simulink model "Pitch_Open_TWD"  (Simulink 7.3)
settings: Solver=ode45  StartTime=0.0  StopTime=20  RelTol=1e-3
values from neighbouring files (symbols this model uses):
  Aac = [    [actuator_srb.m]    (also in actuator_ssme.m; actuators_5s.m; actuators_5z.m)
  Bac = [    [actuator_srb.m]    (also in actuator_ssme.m; actuators_5s.m; actuators_5z.m)
  Cac = [    [actuator_srb.m]    (also in actuator_ssme.m; actuators_5s.m; actuators_5z.m)
  Dac = [    [actuator_srb.m]    (also in actuator_ssme.m; actuators_5s.m; actuators_5z.m)
undefined symbols (not defined in the file or in its folder): Afs, Asb, Atw, Bfs, Bsb, Btw, Cfs, Csb, Ctw, Dfs, Dsb, Dtw

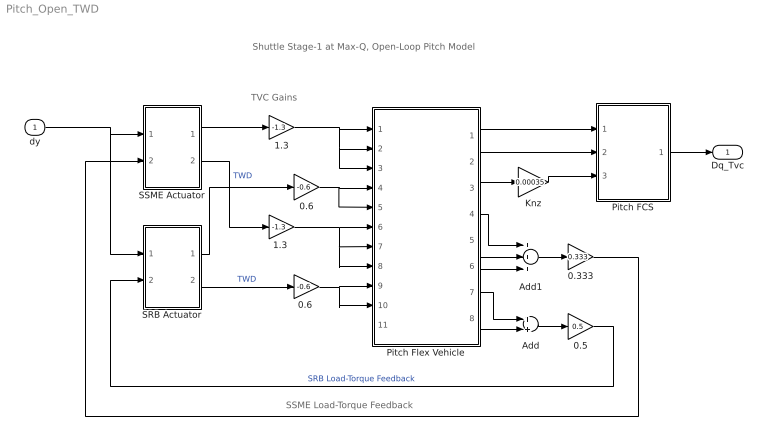
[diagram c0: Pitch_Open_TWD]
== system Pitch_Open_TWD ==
  note: SSME Load-Torque Feedback
  note: TVC Gains
  note: Shuttle Stage-1 at Max-Q, Open-Loop Pitch Model
  dy : Inport  OutDataType=sfix(16)  OutScaling=2^0
  0.333 : Gain  Gain=0.333  ParameterDataType=sfix(16)  ParameterScaling=2^0  OutDataType=sfix(16)  OutScaling=2^0
  0.5 : Gain  Gain=0.5  ParameterDataType=sfix(16)  ParameterScaling=2^0  OutDataType=sfix(16)  OutScaling=2^0
  0.6 : Gain  Gain=-0.6  ParameterDataType=sfix(16)  ParameterScaling=2^0  OutDataType=sfix(16)  OutScaling=2^0
  "0.6 " : Gain  Gain=-0.6  ParameterDataType=sfix(16)  ParameterScaling=2^0  OutDataType=sfix(16)  OutScaling=2^0
  1.3 : Gain  Gain=-1.3  ParameterDataType=sfix(16)  ParameterScaling=2^0  OutDataType=sfix(16)  OutScaling=2^0
  "1.3 " : Gain  Gain=-1.3  ParameterDataType=sfix(16)  ParameterScaling=2^0  OutDataType=sfix(16)  OutScaling=2^0
  Add : Sum  OutDataType=sfix(16)  OutScaling=2^-10
  Add1 : Sum  Inputs=+++  OutDataType=sfix(16)  OutScaling=2^-10
  Knz : Gain  Gain=0.00035  ParameterDataType=sfix(16)  ParameterScaling=2^0  OutDataType=sfix(16)  OutScaling=2^0
  Pitch FCS : Subsystem
  Pitch Flex Vehicle : Subsystem
  SRB Actuator : Subsystem
  SSME Actuator : Subsystem
  Dq_Tvc : Outport  OutDataType=sfix(16)  OutScaling=2^0
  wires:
  SSME Actuator/1(dy) -> 1.3/1
  dy/1 -> SSME Actuator/1(dy-com), SRB Actuator/1(dy-com)
  1.3/1 -> Pitch Flex Vehicle/1(dy1), Pitch Flex Vehicle/2(dy2), Pitch Flex Vehicle/3(dy3)
  0.6/1 -> Pitch Flex Vehicle/4(dy4), Pitch Flex Vehicle/5(dy5)
  SSME Actuator/2(dy-dd) -> "1.3 "/1  "TWD"
  "1.3 "/1 -> Pitch Flex Vehicle/6(dydd1), Pitch Flex Vehicle/7(dydd2), Pitch Flex Vehicle/8(dydd3)
  "0.6 "/1 -> Pitch Flex Vehicle/9(dydd4), Pitch Flex Vehicle/10(dydd5)
  Pitch Flex Vehicle/1(theta) -> Pitch FCS/1(theta)
  Pitch Flex Vehicle/2(q-rb) -> Pitch FCS/2(q)
  Pitch Flex Vehicle/3(Nz) -> Knz/1
  Knz/1 -> Pitch FCS/3(Nz)
  SRB Actuator/1(dy) -> 0.6/1
  SRB Actuator/2(dy-dd) -> "0.6 "/1  "TWD"
  Pitch Flex Vehicle/7(TLy4) -> Add/1
  Pitch Flex Vehicle/8(TLy5) -> Add/2
  Add/1 -> 0.5/1
  0.5/1 -> SRB Actuator/2(TL)  "SRB Load-Torque Feedback"
  Add1/1 -> 0.333/1
  Pitch Flex Vehicle/6(TLy3) -> Add1/3
  Pitch Flex Vehicle/5(TLy2) -> Add1/2
  Pitch Flex Vehicle/4(TLy1) -> Add1/1
  0.333/1 -> SSME Actuator/2(TL)
  Pitch FCS/1(DQ_TVC) -> Dq_Tvc/1

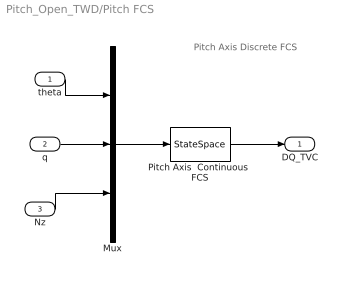
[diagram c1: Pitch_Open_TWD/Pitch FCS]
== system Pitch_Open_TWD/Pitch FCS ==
  note: Pitch Axis Discrete FCS
  theta : Inport  OutDataType=sfix(16)  OutScaling=2^0
  q : Inport  Port=2  OutDataType=sfix(16)  OutScaling=2^0
  Nz : Inport  Port=3  OutDataType=sfix(16)  OutScaling=2^0
  Mux : Mux  Inputs=3
  Pitch Axis  Continuous  FCS : StateSpace  A=Afs  B=Bfs  C=Cfs  D=Dfs
  DQ_TVC : Outport  OutDataType=sfix(16)  OutScaling=2^0
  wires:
  Pitch Axis  Continuous  FCS/1 -> DQ_TVC/1
  theta/1 -> Mux/1
  q/1 -> Mux/2
  Nz/1 -> Mux/3
  Mux/1 -> Pitch Axis  Continuous  FCS/1

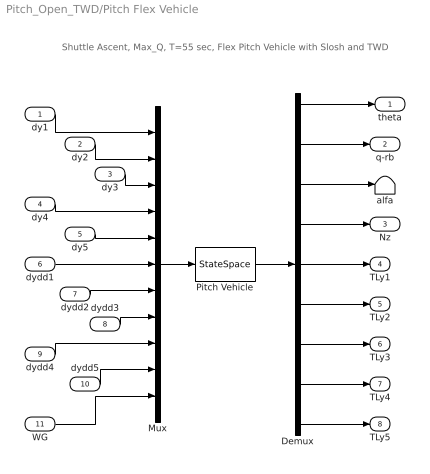
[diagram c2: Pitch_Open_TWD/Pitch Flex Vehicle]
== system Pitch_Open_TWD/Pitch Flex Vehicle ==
  note: Shuttle Ascent, Max_Q, T=55 sec, Flex Pitch Vehicle with Slosh and TWD
  dy1 : Inport  OutDataType=sfix(16)  OutScaling=2^0
  dy2 : Inport  Port=2  OutDataType=sfix(16)  OutScaling=2^0
  dy3 : Inport  Port=3  OutDataType=sfix(16)  OutScaling=2^0
  dy4 : Inport  Port=4  OutDataType=sfix(16)  OutScaling=2^0
  dy5 : Inport  Port=5  OutDataType=sfix(16)  OutScaling=2^0
  dydd1 : Inport  Port=6  OutDataType=sfix(16)  OutScaling=2^0
  dydd2 : Inport  Port=7  OutDataType=sfix(16)  OutScaling=2^0
  dydd3 : Inport  Port=8  OutDataType=sfix(16)  OutScaling=2^0
  dydd4 : Inport  Port=9  OutDataType=sfix(16)  OutScaling=2^0
  dydd5 : Inport  Port=10  OutDataType=sfix(16)  OutScaling=2^0
  WG : Inport  Port=11  OutDataType=sfix(16)  OutScaling=2^0
  Demux : Demux  Outputs=9
  Mux : Mux  Inputs=11
  Pitch Vehicle : StateSpace  A=Atw  B=Btw  C=Ctw  D=Dtw
  alfa : Terminator
  theta : Outport  OutDataType=sfix(16)  OutScaling=2^0
  q-rb : Outport  Port=2  OutDataType=sfix(16)  OutScaling=2^0
  Nz : Outport  Port=3  OutDataType=sfix(16)  OutScaling=2^0
  TLy1 : Outport  Port=4  OutDataType=sfix(16)  OutScaling=2^0
  TLy2 : Outport  Port=5  OutDataType=sfix(16)  OutScaling=2^0
  TLy3 : Outport  Port=6  OutDataType=sfix(16)  OutScaling=2^0
  TLy4 : Outport  Port=7  OutDataType=sfix(16)  OutScaling=2^0
  TLy5 : Outport  Port=8  OutDataType=sfix(16)  OutScaling=2^0
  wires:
  Pitch Vehicle/1 -> Demux/1
  Mux/1 -> Pitch Vehicle/1
  Demux/3 -> alfa/1
  dy1/1 -> Mux/1
  dy2/1 -> Mux/2
  dy3/1 -> Mux/3
  dy4/1 -> Mux/4
  dy5/1 -> Mux/5
  dydd1/1 -> Mux/6
  dydd2/1 -> Mux/7
  dydd3/1 -> Mux/8
  dydd4/1 -> Mux/9
  dydd5/1 -> Mux/10
  WG/1 -> Mux/11
  Demux/1 -> theta/1
  Demux/4 -> Nz/1
  Demux/5 -> TLy1/1
  Demux/6 -> TLy2/1
  Demux/7 -> TLy3/1
  Demux/8 -> TLy4/1
  Demux/9 -> TLy5/1
  Demux/2 -> q-rb/1

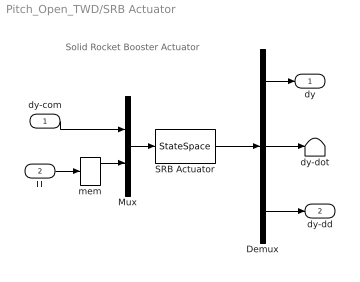
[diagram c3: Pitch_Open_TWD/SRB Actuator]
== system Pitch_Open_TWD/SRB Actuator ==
  note: Solid Rocket Booster Actuator
  dy-com : Inport  PortDimensions=1  OutDataType=sfix(16)  OutScaling=2^0
  TL : Inport  Port=2  OutDataType=sfix(16)  OutScaling=2^0
  Demux : Demux  Outputs=3
  Mux : Mux  Inputs=2
  SRB Actuator : StateSpace  A=Asb  B=Bsb  C=Csb  D=Dsb
  dy-dot : Terminator
  mem : Memory
  dy : Outport  OutDataType=sfix(16)  OutScaling=2^0
  dy-dd : Outport  Port=2  OutDataType=sfix(16)  OutScaling=2^0
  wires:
  SRB Actuator/1 -> Demux/1
  Mux/1 -> SRB Actuator/1
  Demux/1 -> dy/1
  dy-com/1 -> Mux/1
  TL/1 -> mem/1
  Demux/2 -> dy-dot/1
  Demux/3 -> dy-dd/1
  mem/1 -> Mux/2

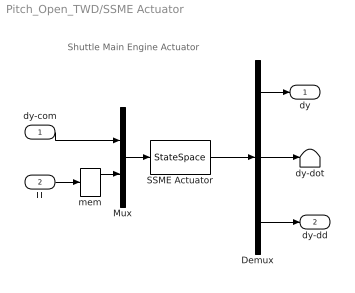
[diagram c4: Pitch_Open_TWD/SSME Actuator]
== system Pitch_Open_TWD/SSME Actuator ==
  note: Shuttle Main Engine Actuator
  dy-com : Inport  PortDimensions=1  OutDataType=sfix(16)  OutScaling=2^0
  TL : Inport  Port=2  OutDataType=sfix(16)  OutScaling=2^0
  Demux : Demux  Outputs=3
  Mux : Mux  Inputs=2
  SSME Actuator : StateSpace  A=Aac  B=Bac  C=Cac  D=Dac
  dy-dot : Terminator
  mem : Memory
  dy : Outport  OutDataType=sfix(16)  OutScaling=2^0
  dy-dd : Outport  Port=2  OutDataType=sfix(16)  OutScaling=2^0
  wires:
  SSME Actuator/1 -> Demux/1
  Mux/1 -> SSME Actuator/1
  Demux/1 -> dy/1
  dy-com/1 -> Mux/1
  TL/1 -> mem/1
  Demux/2 -> dy-dot/1
  Demux/3 -> dy-dd/1
  mem/1 -> Mux/2
